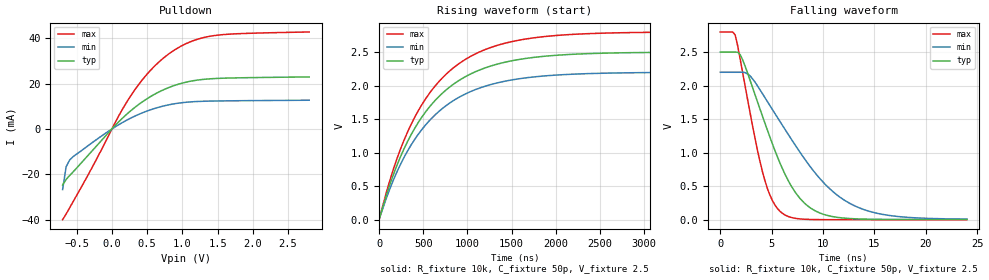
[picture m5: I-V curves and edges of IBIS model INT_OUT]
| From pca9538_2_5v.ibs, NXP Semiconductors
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[Model]   INT_OUT
Model_type Open_drain
Vref=2.5
Vmeas=1.25
Rref=10k
Cref=50p
C_comp   5.2p   5p   5.4p
[Temperature Range] 27   85   -40
[Voltage Range]   2.5   2.2   2.8
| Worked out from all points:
|   slope of the pulldown table from 0 to 0.375 V, typ, clamps not added: 35.1 ohm
|   falling waveform, R_fixture 10k, C_fixture 50p, V_fixture 2.5: 20-80 % time 3.84ns typ, 6.17ns min, 2.27ns max; typ from 2.5 V to 0.007 V
|   rising waveform, R_fixture 10k, C_fixture 50p, V_fixture 2.5: 20-80 % time 704ns typ, 705ns min, 702ns max; typ from 0.007 V to 2.5 V
[Pulldown]
-700mV    -24.78mA   -26.76mA   -40.07mA
-650mV    -22.28mA   -16.7mA    -37.53mA
-600mV    -20.55mA   -13.7mA    -34.82mA
-550mV    -18.94mA   -12.2mA    -32.07mA
-250mV    -8.603mA   -5.373mA   -15.2mA
100mV     3.26mA     1.947mA    5.975mA
250mV     7.594mA    4.531mA    13.84mA
500mV     13.39mA    7.941mA    24.26mA
800mV     18.21mA    10.62mA    32.99mA
1.1V      20.99mA    11.92mA    38.33mA
1.4V      22.16mA    12.31mA    40.99mA
2.8V      22.98mA    12.69mA    42.84mA
[Falling Waveform]
R_fixture=10k
C_fixture=50p
V_fixture=2.5
V_fixture_min=2.2
V_fixture_max=2.8
0s        2.5V       2.2V       2.8V
1.455ns   2.5V       2.2V       2.753V
2.182ns   2.383V     2.2V       2.19V
4.121ns   1.54V      1.877V     707.7mV
5.091ns   1.127V     1.641V     283.5mV
6.061ns   761.2mV    1.407V     97.85mV
8.727ns   183.9mV    799.9mV    7.812mV
12.85ns   19.6mV     228.2mV    4.505mV
16.73ns   8.305mV    61.83mV    4.487mV
24ns      7.379mV    13.82mV    4.487mV
[Rising Waveform]
R_fixture=10k
C_fixture=50p
V_fixture=2.5
V_fixture_min=2.2
V_fixture_max=2.8
0s        7.369mV    10.85mV    4.487mV
121.2ns   524.8mV    462.6mV    587.5mV
202ns     814.4mV    716.8mV    912.7mV
323.2ns   1.172V     1.031V     1.314V
444.4ns   1.453V     1.278V     1.629V
727.3ns   1.9V       1.671V     2.13V
1.051us   2.183V     1.92V      2.446V
1.414us   2.345V     2.063V     2.627V
1.939us   2.445V     2.151V     2.739V
4us       2.499V     2.199V     2.799V
[Ramp]
R_load=10k
dV/dt_r   1.391E+0/1.002E-8   1.351E+0/1.044E-8   1.428E+0/9.349E-9
dV/dt_f   1.496E+0/1.653E-10   1.493E+0/3.277E-10   1.498E+0/1.179E-10
|[End   INT_OUT
